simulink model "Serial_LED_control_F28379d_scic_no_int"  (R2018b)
settings: Solver=FixedStepDiscrete  StartTime=0.0  StopTime=inf  RelTol=1e-3  EnableMultiTasking=on
PostLoadFcn:
  | c2000demoscallback(1)
libraries: c2837xDlib x4, c280xlib x2

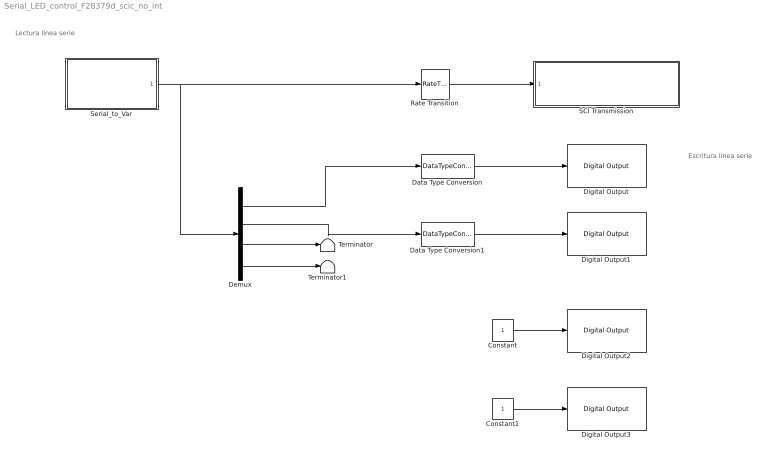
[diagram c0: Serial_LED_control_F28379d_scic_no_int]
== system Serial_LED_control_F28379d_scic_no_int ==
  note: Lectura línea serie
  note: Escritura línea serie
  Constant : Constant
  Constant1 : Constant
  Data Type Conversion : DataTypeConversion
  Data Type Conversion1 : DataTypeConversion
  Demux : Demux
  Digital Output : c2837xDlib/Digital Output  GPIO_Number=GPIO24~GPIO31  GPIO_Bit0=off  GPIO_BIT0_Toggle=off  GPIO_Bit1=off  GPIO_BIT1_Toggle=off  GPIO_Bit2=off  GPIO_BIT2_Toggle=off  GPIO_Bit3=off  GPIO_BIT3_Toggle=off  GPIO_Bit4=off  GPIO_BIT4_Toggle=off  GPIO_Bit5=off  GPIO_BIT5_Toggle=off  GPIO_Bit6=off  GPIO_BIT6_Toggle=off  GPIO_Bit7=on  GPIO_BIT7_Toggle=off
  Digital Output1 : c2837xDlib/Digital Output  GPIO_Number=GPIO32~GPIO39  GPIO_Bit0=off  GPIO_BIT0_Toggle=off  GPIO_Bit1=off  GPIO_BIT1_Toggle=off  GPIO_Bit2=on  GPIO_BIT2_Toggle=off  GPIO_Bit3=off  GPIO_BIT3_Toggle=off  GPIO_Bit4=off  GPIO_BIT4_Toggle=off  GPIO_Bit5=off  GPIO_BIT5_Toggle=off  GPIO_Bit6=off  GPIO_BIT6_Toggle=off  GPIO_Bit7=off  GPIO_BIT7_Toggle=off
  Digital Output2 : c2837xDlib/Digital Output  GPIO_Number=GPIO64~GPIO71  GPIO_Bit0=off  GPIO_BIT0_Toggle=off  GPIO_Bit1=off  GPIO_BIT1_Toggle=off  GPIO_Bit2=on  GPIO_BIT2_Toggle=off  GPIO_Bit3=off  GPIO_BIT3_Toggle=off  GPIO_Bit4=off  GPIO_BIT4_Toggle=off  GPIO_Bit5=off  GPIO_BIT5_Toggle=off  GPIO_Bit6=off  GPIO_BIT6_Toggle=off  GPIO_Bit7=off  GPIO_BIT7_Toggle=off
  Digital Output3 : c2837xDlib/Digital Output  GPIO_Number=GPIO128~GPIO135  GPIO_Bit0=off  GPIO_BIT0_Toggle=off  GPIO_Bit1=off  GPIO_BIT1_Toggle=off  GPIO_Bit2=off  GPIO_BIT2_Toggle=off  GPIO_Bit3=on  GPIO_BIT3_Toggle=off  GPIO_Bit4=off  GPIO_BIT4_Toggle=off  GPIO_Bit5=off  GPIO_BIT5_Toggle=off  GPIO_Bit6=off  GPIO_BIT6_Toggle=off  GPIO_Bit7=off  GPIO_BIT7_Toggle=off
  Rate Transition : RateTransition  Deterministic=off
  SCI Transmission : Subsystem
  Serial_to_Var : Subsystem
  Terminator : Terminator
  Terminator1 : Terminator
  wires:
  Rate Transition/1 -> SCI Transmission/1(In1)
  Serial_to_Var/1(Serial_to_var) -> Demux/1, Rate Transition/1
  Demux/1 -> Data Type Conversion/1
  Demux/2 -> Data Type Conversion1/1
  Demux/3 -> Terminator/1
  Demux/4 -> Terminator1/1
  Data Type Conversion/1 -> Digital Output/1
  Data Type Conversion1/1 -> Digital Output1/1
  Constant/1 -> Digital Output2/1
  Constant1/1 -> Digital Output3/1

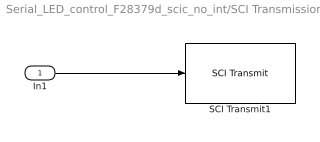
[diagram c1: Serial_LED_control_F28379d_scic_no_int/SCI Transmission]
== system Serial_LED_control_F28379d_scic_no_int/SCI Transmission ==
  In1 : Inport
  SCI Transmit1 : c280xlib/SCI Transmit  sciModule=C  dataHead='S'  dataTail='E'  postInterrupt=off  numFifo=1
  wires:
  In1/1 -> SCI Transmit1/1

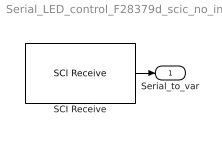
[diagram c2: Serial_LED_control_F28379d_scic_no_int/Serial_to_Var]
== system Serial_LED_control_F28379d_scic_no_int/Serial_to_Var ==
  SCI Receive : c280xlib/SCI Receive  sciModule=C  dataHead='S'  dataTail='E'  dataType=uint8  dataDim=4  initValue=1  errOption=Output the last received value  errValue=0  sampleTime=0.1  outputStatus=off  postInterrupt=on  numFifo=0
  Serial_to_var : Outport
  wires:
  SCI Receive/1 -> Serial_to_var/1
